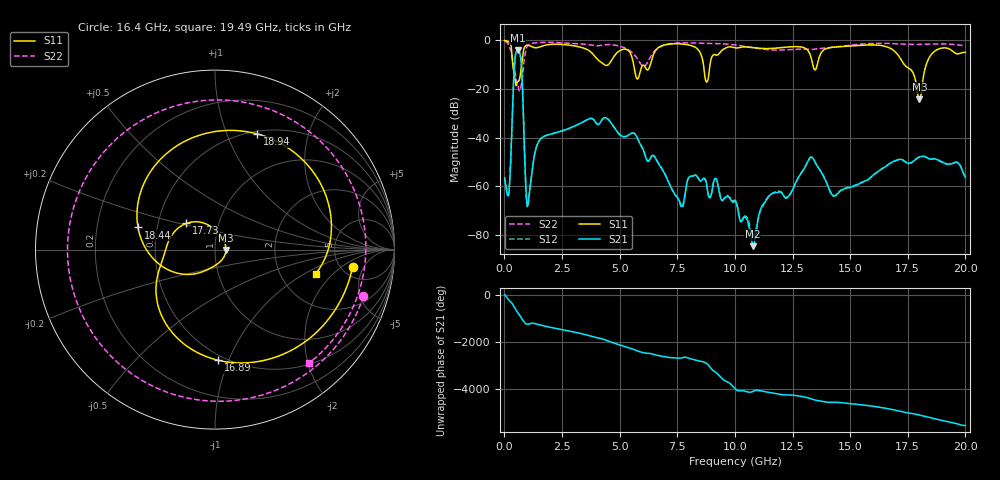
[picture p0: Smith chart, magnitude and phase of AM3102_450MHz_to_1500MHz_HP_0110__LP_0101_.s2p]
!Agilent Technologies,E8364B,MY43040894,A.07.50.67
!Agilent E8364B: A.07.50.67
!Date: Thursday, January 11, 2018 05:46:53
!Correction: S11(Full 2 Port(1,2))
!S21(Full 2 Port(1,2))
!S12(Full 2 Port(1,2))
!S22(Full 2 Port(1,2))
!S2P File: Measurements: S11, S21, S12, S22:
# Hz S  dB  R 50
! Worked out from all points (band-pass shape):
!   1601 points, 10 MHz to 20 GHz, reference 50 ohm
!   highest |S21| = -4.14 dB at 572.2 MHz (marker M1); lowest = -84.6 dB at 10.78 GHz (marker M2)
!   |S21| within 3 dB of the highest: 466.9 MHz to 707.3 MHz (240.4 MHz wide, 40.9 % of centre)
!   lowest |S11| = -24.3 dB at 18 GHz (marker M3), VSWR 1.13, Z = 56.5 - j0.271 ohm
!   |S11| at or under -10 dB: 364.3 MHz to 748.2 MHz (383.9 MHz wide, 69 % of centre); 5.606 GHz to 6.332 GHz (725.9 MHz wide, 12.2 % of centre); 17.35 GHz to 18.3 GHz (948.5 MHz wide, 5.32 % of centre)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
!   |S22| runs from -20.8 to -0.4 dB; largest |S21 - S12| = 0.0026
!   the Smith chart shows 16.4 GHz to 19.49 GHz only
!   S11 on the Smith chart (normalised r, x): 16.4 GHz: 6.29, -3.04; 16.89 GHz: 0.46, -0.92; 17.73 GHz: 0.70, +0.21; 18.44 GHz: 0.39, +0.12; 18.94 GHz: 0.53, +1.29; 19.49 GHz: 3.17, -1.28
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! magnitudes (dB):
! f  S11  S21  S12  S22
! 10 MHz  -0.1  -57.1  -56.1  -0.4
! 197.4 MHz  -0.7  -62.7  -61.9  -2.5
! 572.2 MHz  -16.9  -4.1  -4.1  -18.0
! 722.1 MHz  -11.9  -8.3  -8.3  -19.0
! 1.022 GHz  -2.0  -67.6  -68.6  -2.1
! 1.534 GHz  -2.7  -40.9  -40.9  -0.9
! 3.346 GHz  -3.0  -33.9  -33.9  -1.5
! 6.682 GHz  -3.0  -50.6  -50.5  -3.1
! 8.781 GHz  -17.1  -59.7  -59.7  -1.2
! 10.01 GHz  -3.1  -66.1  -65.8  -1.9
! 10.78 GHz  -3.0  -84.6  -80.2  -3.0
! 13.34 GHz  -8.4  -48.1  -48.0  -3.8
! 14.29 GHz  -2.8  -63.9  -64.0  -2.8
! 16.4 GHz  -2.2  -52.7  -52.7  -1.2
! 16.68 GHz  -3.0  -50.9  -50.9  -1.3
! 16.89 GHz  -4.2  -49.8  -49.7  -1.4
! 17.73 GHz  -13.3  -49.8  -49.8  -1.7
! 18 GHz  -24.3  -48.0  -47.9  -1.7
! 18.44 GHz  -7.0  -48.7  -48.8  -1.6
! 18.94 GHz  -3.3  -49.7  -49.9  -1.5
! 19.49 GHz  -4.8  -50.4  -50.5  -1.7
! 20 GHz  -5.0  -56.2  -55.9  -2.2
